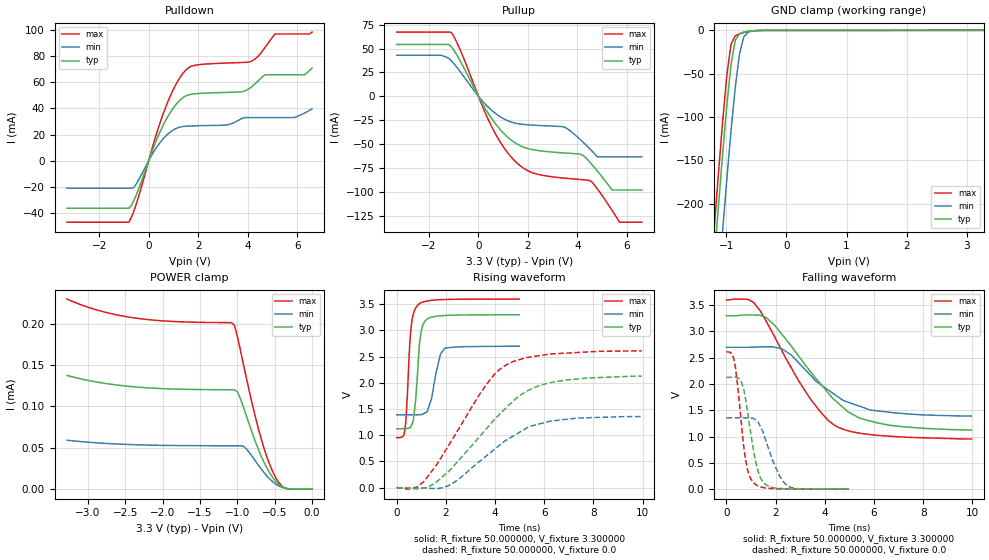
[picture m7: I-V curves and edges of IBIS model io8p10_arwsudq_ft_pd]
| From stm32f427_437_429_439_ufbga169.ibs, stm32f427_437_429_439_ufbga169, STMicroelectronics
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|   Model io8p10_arwsudq_ft_pd
[Model]  io8p10_arwsudq_ft_pd
Model_type I/O
Polarity   Non-Inverting
Enable   Active-Low
Vinl =   0.990000V
Vinh =   2.310000V
Vmeas =  1.650000V
Cref =   40.000000pF
Rref =   100.000000M
Vref =   0.0V
C_comp   2.905500pF   2.826300pF   2.987900pF
[Temperature Range]   25.000000   0.125000k   -40.000000
[Pullup Reference]   3.300000V   2.700000V   3.600000V
[Pulldown Reference]   0.0V   0.0V   0.0V
[POWER Clamp Reference]   3.300000V   2.700000V   3.600000V
[GND Clamp Reference]   0.0V   0.0V   0.0V
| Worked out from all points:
|   slope of the pulldown table from 0 to 0.495 V, typ, clamps not added: 20.9 ohm
|   slope of the pullup table from 0 to 0.495 V, typ, clamps not added: 22.6 ohm
|   GND clamp passes 1 mA (typ) near -0.62 V on its own axis
|   rising waveform, R_fixture 50.000000, V_fixture 3.300000: 20-80 % time 215ps typ, 342ps min, 189ps max; typ from 1.12 V to 3.3 V
|   rising waveform, R_fixture 50.000000, V_fixture 0.0: 20-80 % time 2.52ns typ, 2.31ns min, 2.11ns max; typ from 0 V to 2.13 V
|   falling waveform, R_fixture 50.000000, V_fixture 3.300000: 20-80 % time 2.33ns typ, 2.09ns min, 2.04ns max; typ from 3.3 V to 1.12 V
|   falling waveform, R_fixture 50.000000, V_fixture 0.0: 20-80 % time 460ps typ, 654ps min, 368ps max; typ from 2.13 V to 0 V
[Pulldown]
|Voltage   I(typ)   I(min)   I(max)
-3.3V     -36.4mA    -21.07mA   -47.09mA
-800mV    -36.4mA    -21.07mA   -47.09mA
-600mV    -30.5mA    -20.54mA   -38.69mA
700mV     31.4mA     19.11mA    41.71mA
1.2V      45.15mA    25.37mA    61.75mA
1.6V      50.35mA    26.5mA     71.06mA
3.1V      52.27mA    27.26mA    74.75mA
4.1V      55.71mA    33.04mA    75.8mA
4.7V      65.8mA     33.04mA    86.69mA
5.1V      65.8mA     33.04mA    97.03mA
6.3V      65.87mA    36.5mA     97.03mA
6.6V      70.92mA    39.71mA    98.48mA
[Pullup]
|Voltage   I(typ)   I(min)   I(max)
-3.3V     54.25mA    42.91mA    67.2mA
-1.1V     52mA       37.31mA    66.9mA
500mV     -22.07mA   -14mA      -30.03mA
1.5V      -49.1mA    -28.3mA    -68.56mA
2.2V      -56.04mA   -30.32mA   -80.35mA
3.5V      -59.53mA   -32.66mA   -85.92mA
4.2V      -61.44mA   -47.49mA   -87.46mA
4.5V      -69.08mA   -55.13mA   -88.39mA
4.8V      -78.24mA   -63.5mA    -96.88mA
5.4V      -98.3mA    -63.5mA    -119.6mA
5.7V      -98.3mA    -63.5mA    -132mA
6.6V      -98.3mA    -63.5mA    -132mA
[GND_clamp]
|Voltage   I(typ)   I(min)   I(max)
-3.3V     -2.317A    -2.396A    -2.29A
-1.2V     -266mA     -356.3mA   -228.4mA
-1.13V    -203.2mA   -293mA     -165.3mA
-1.06V    -142.7mA   -231.3mA   -105.2mA
-990mV    -86.51mA   -171.7mA   -51.78mA
-920mV    -39.3mA    -115.7mA   -15.95mA
-850mV    -11.38mA   -65.76mA   -6.112mA
-780mV    -3.842mA   -27.55mA   -3.895mA
-710mV    -2.102mA   -7.755mA   -2.396mA
-640mV    -1.159mA   -2.138mA   -1.234mA
-570mV    -535.1uA   -809uA     -490.4uA
3.28V     81.28uA    57.87uA    93.98uA
[POWER_clamp]
|Voltage   I(typ)   I(min)   I(max)
-3.28V    137.3uA    59.14uA    229.6uA
-2.36V    123.4uA    53.65uA    206.6uA
-1.08V    120.1uA    52.41uA    201.1uA
-1.04V    120uA      52.41uA    198uA
-1V       117.7uA    52.4uA     184.5uA
-920mV    99.46uA    51.91uA    151.2uA
-720mV    48.42uA    29.12uA    73.51uA
-600mV    24.82uA    15.47uA    37.72uA
-520mV    13.1uA     8.45uA     19.84uA
-440mV    5.058uA    3.61uA     7.276uA
-360mV    1.193uA    1.129uA    1.311uA
0V        0A         0A         0A
[Ramp]
| variable   typ   min   max
dV/dt_r  1.26636/2.51443n   0.81090/2.30875n   1.56449/2.11219n
dV/dt_f  1.28256/2.32084n   0.77658/2.07713n   1.57441/2.03993n
R_load = 50.000000
[Rising Waveform]
R_fixture= 50.000000
V_fixture= 3.300000
V_fixture_min= 2.700000
V_fixture_max= 3.600000
|time   V(typ)   V(min)   V(max)
0s        1.123V     1.391V     953.9mV
310.3ps   1.125V     1.391V     1.043V
380.4ps   1.127V     1.391V     1.33V
570.6ps   1.158V     1.391V     2.995V
670.7ps   1.271V     1.39V      3.305V
830.8ps   2.081V     1.391V     3.468V
981ps     2.942V     1.393V     3.525V
1.251ns   3.221V     1.468V     3.562V
1.962ns   3.284V     2.663V     3.589V
4.985ns   3.299V     2.699V     3.598V
[Rising Waveform]
R_fixture= 50.000000
V_fixture= 0.0
V_fixture_min= 0.0
V_fixture_max= 0.0
|time   V(typ)   V(min)   V(max)
0s        349uV      197.8uV    665.1uV
580.6ps   -7.683mV   200.6uV    -18.73mV
1.101ns   -5.297mV   -2.568mV   115.5mV
1.522ns   70.65mV    -16.64mV   376.7mV
2.142ns   324.6mV    46.06mV    830.2mV
3.664ns   1.132V     613.6mV    1.978V
4.505ns   1.549V     920.6mV    2.355V
5.285ns   1.841V     1.137V     2.481V
6.206ns   1.999V     1.266V     2.548V
9.97ns    2.127V     1.357V     2.611V
[Falling Waveform]
R_fixture= 50.000000
V_fixture= 3.300000
V_fixture_min= 2.700000
V_fixture_max= 3.600000
|time   V(typ)   V(min)   V(max)
0s        3.299V     2.699V     3.598V
900.9ps   3.314V     2.699V     3.605V
1.101ns   3.313V     2.701V     3.554V
1.602ns   3.269V     2.71V      3.205V
2.262ns   2.944V     2.669V     2.628V
3.423ns   2.23V      2.165V     1.71V
4.444ns   1.678V     1.787V     1.203V
5.445ns   1.346V     1.573V     1.063V
6.126ns   1.263V     1.49V      1.025V
9.97ns    1.123V     1.391V     953.9mV
[Falling Waveform]
R_fixture= 50.000000
V_fixture= 0.0
V_fixture_min= 0.0
V_fixture_max= 0.0
|time   V(typ)   V(min)   V(max)
0s        2.127V     1.357V     2.611V
300.3ps   2.128V     1.357V     2.481V
460.5ps   2.117V     1.357V     1.951V
620.6ps   2.021V     1.357V     1.188V
850.9ps   1.499V     1.359V     388.6mV
1.091ns   768.6mV    1.349V     130.6mV
1.481ns   140mV      1.089V     33.42mV
2.152ns   14.65mV    256.5mV    5.626mV
2.452ns   6.534mV    75.27mV    3.972mV
4.985ns   349uV      197.8uV    665.1uV
